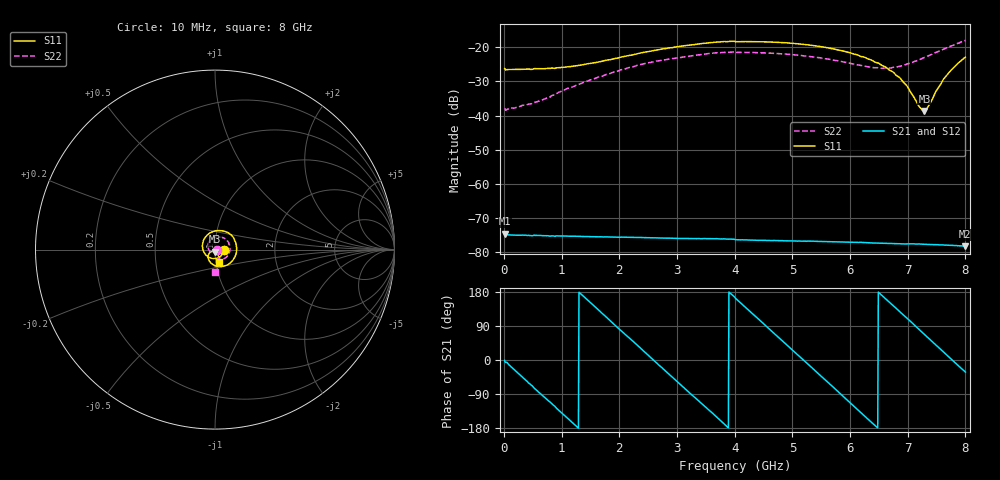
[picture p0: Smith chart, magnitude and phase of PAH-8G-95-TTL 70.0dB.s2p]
! MTS Systemtechnik GmbH
! S-Parameters
! Model: PAH-8G/95-TTL
! Attenuation Step: 70.0dB
! Rohde & Schwarz ZVB8 2Ports - Version 4.11 - 1145.1010k08 SN: 100119
! S2P File Measurements:
! S11 S21 S12 S22
# HZ  S  DB  R  50.00
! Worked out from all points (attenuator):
!   800 points, 10 MHz to 8 GHz, reference 50 ohm
!   highest |S21| = -74.61 dB at 10 MHz (marker M1); lowest = -78.2 dB at 7.99 GHz (marker M2)
!   lowest |S11| = -38.7 dB at 7.29 GHz (marker M3), VSWR 1.02, Z = 49.8 - j1.14 ohm
!   |S11| at or under -10 dB: start of sweep to end of sweep
!   |S22| runs from -38.4 to -18.0 dB; largest |S21 - S12| = 2.7e-06
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1e7  -26.22 -2.6  -74.61 -1.4  -74.51 -1.2  -37.89 -9.4
5.1e8  -26.32 -49.3  -75.07 -72.3  -75.11 -72.0  -36.28 -70.7
1.35e9  -25.16 -131.9  -75.41 172.0  -75.41 172.0  -30.49 -160.9
2.05e9  -22.78 165.3  -75.63 74.7  -75.62 74.8  -26.50 144.7
2.68e9  -20.68 116.7  -75.86 -12.8  -75.84 -12.2  -23.95 103.7
3.39e9  -18.98 68.5  -76.04 -110.1  -76.08 -110.4  -22.16 60.9
4.01e9  -18.34 27.7  -76.34 163.3  -76.35 163.4  -21.48 25.5
4.63e9  -18.43 -11.8  -76.61 77.6  -76.61 77.5  -21.68 -7.9
5.34e9  -19.42 -57.4  -76.79 -20.5  -76.81 -20.4  -22.75 -42.7
6.11e9  -22.10 -107.3  -77.11 -128.1  -77.14 -127.8  -25.04 -68.7
6.49e9  -24.61 -131.2  -77.36 179.2  -77.37 179.1  -25.99 -71.2
6.67e9  -26.50 -140.6  -77.44 154.1  -77.46 154.2  -26.12 -69.6
6.89e9  -29.45 -148.6  -77.56 123.6  -77.59 123.6  -25.42 -67.6
7e9  -31.62 -149.3  -77.59 108.6  -77.60 108.7  -24.81 -66.9
7.2e9  -37.37 -131.1  -77.62 80.3  -77.63 80.3  -23.65 -67.7
7.29e9  -38.66 -101.0  -77.68 67.5  -77.72 67.3  -22.96 -68.6
7.36e9  -37.16 -79.6  -77.72 57.6  -77.78 57.7  -22.44 -69.5
7.5e9  -32.60 -60.7  -77.84 38.1  -77.86 37.9  -21.40 -72.5
7.65e9  -28.70 -59.7  -77.96 17.1  -77.94 17.2  -20.35 -77.1
7.85e9  -24.99 -67.0  -78.06 -10.9  -78.13 -10.8  -18.92 -84.2
7.99e9  -23.01 -73.6  -78.25 -30.5  -78.21 -30.2  -18.02 -89.8
8e9  -22.89 -74.1  -78.24 -31.9  -78.24 -31.4  -17.98 -90.4
